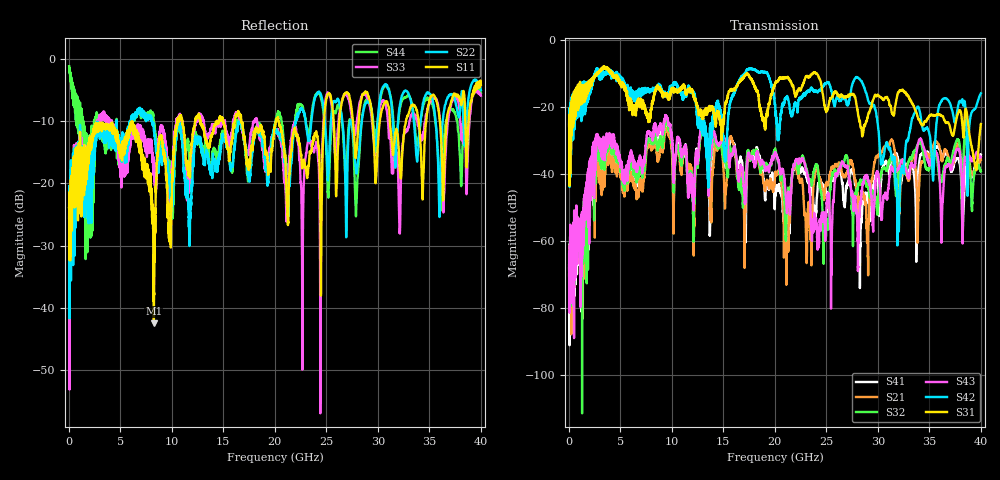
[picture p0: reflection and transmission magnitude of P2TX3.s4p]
!Agilent Technologies,N5245A,MY49151084,A.09.20.08
!Agilent N5245A: A.09.20.08
!Date: Thursday, March 01, 2012 13:22:45
!Correction: S11(Full 4 Port(1,2,3,4))
!S12(Full 4 Port(1,2,3,4))
!S13(Full 4 Port(1,2,3,4))
!S14(Full 4 Port(1,2,3,4))
!S21(Full 4 Port(1,2,3,4))
!S22(Full 4 Port(1,2,3,4))
!S23(Full 4 Port(1,2,3,4))
!S24(Full 4 Port(1,2,3,4))
!S31(Full 4 Port(1,2,3,4))
!S32(Full 4 Port(1,2,3,4))
!S33(Full 4 Port(1,2,3,4))
!S34(Full 4 Port(1,2,3,4))
!S41(Full 4 Port(1,2,3,4))
!S42(Full 4 Port(1,2,3,4))
!S43(Full 4 Port(1,2,3,4))
!S44(Full 4 Port(1,2,3,4))
!S4P File: Measurements: <S11,S12,S13,S14>,
!<S21,S22,S23,S24>,
!<S31,S32,S33,S34>,
!<S41,S42,S43,S44>:
# Hz S  dB  R 50
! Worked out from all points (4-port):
!   3996 points, 50 MHz to 40 GHz, reference 50 ohm
!   strongest paths, dB at 50 MHz, 10.04 GHz, 20.03 GHz, 30.02 GHz, 40 GHz:
!     S31: -25.6, -15.0, -12.9, -16.5, -25.0
!     S42: -25.0, -13.5, -19.2, -25.7, -15.9
!     S43: -67.1, -30.0, -33.6, -39.6, -34.9
!     S32: -63.9, -31.3, -32.4, -49.6, -39.1
!     S21: -69.9, -34.6, -39.3, -34.6, -35.7
!     S41: -68.1, -33.0, -45.9, -45.0, -34.2
!   lowest |S11| = -42.4 dB at 8.27 GHz (marker M1), VSWR 1.02, Z = 49.3 - j0.324 ohm
!   |S11| at or under -10 dB: start of sweep to 10.55 GHz; 16.76 GHz to 20.11 GHz (3.352 GHz wide, 18.2 % of centre); 20.37 GHz to 24.77 GHz (4.395 GHz wide, 19.5 % of centre)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
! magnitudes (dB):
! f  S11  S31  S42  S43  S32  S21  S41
! 50 MHz  -23.8  -25.6  -25.0  -67.1  -63.9  -69.9  -68.1
! 2.81 GHz  -10.6  -9.6  -8.6  -29.2  -33.0  -36.6  -33.2
! 8.27 GHz  -42.4  -16.5  -14.8  -26.4  -28.9  -30.9  -28.9
! 28.06 GHz  -12.0  -21.6  -11.2  -61.3  -44.2  -47.2  -46.8
! 31.98 GHz  -13.3  -15.5  -49.1  -38.5  -40.5  -41.3  -35.6
! 33.78 GHz  -8.3  -21.8  -20.2  -33.0  -31.9  -44.3  -52.3
! 40 GHz  -4.2  -25.0  -15.9  -34.9  -39.1  -35.7  -34.2
